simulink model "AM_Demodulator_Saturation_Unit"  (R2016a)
settings: Solver=ode3  StartTime=0.0  StopTime=6  FixedStep=1/5000000  RelTol=1e-3
libraries: dsparch4 x1

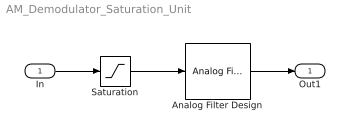
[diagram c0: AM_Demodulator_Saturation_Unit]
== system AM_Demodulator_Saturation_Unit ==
  In : Inport
  Analog Filter Design : dsparch4/Analog Filter Design  method=Butterworth  filttype=Lowpass  N=8  Wlo=45000*2*pi  Whi=80  Rp=2  Rs=40
  Saturation : Saturate  UpperLimit=inf  LowerLimit=0
  Out1 : Outport
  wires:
  In/1 -> Saturation/1
  Analog Filter Design/1 -> Out1/1
  Saturation/1 -> Analog Filter Design/1
